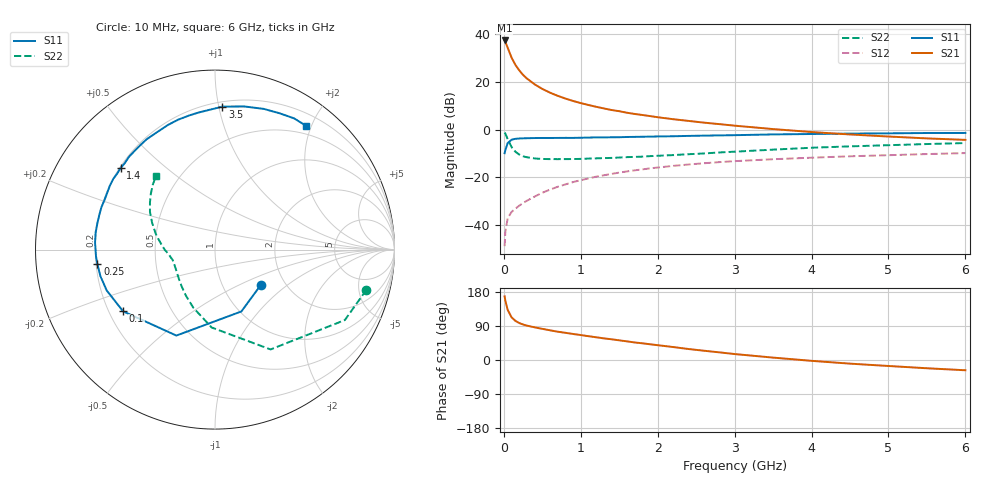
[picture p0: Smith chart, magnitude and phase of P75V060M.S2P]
! SIEMENS Small Signal Semiconductors
! BFP196
! Si NPN RF Bipolar Junction Transistor in SOT143
! VCE = 5 V  IC = 60 mA
! Common Emitter S-Parameters:  May  1996
# GHz  S  MA  R  50
!  f  S11  S21  S12  S22
! GHz  MAG  ANG  MAG  ANG  MAG  ANG  MAG  ANG
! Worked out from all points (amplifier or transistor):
!   36 points, 10 MHz to 6 GHz, reference 50 ohm
!   highest |S21| = 37.5 dB at 10 MHz (marker M1)
!   |S21| within 3 dB of that: start of sweep to 49.2 MHz
!   unconditionally stable (mu >= 1): 442.7 MHz to 4.365 GHz
!   at 250 MHz: K = 0.85, MSG = 26.9 dB, |S12| = -30.8 dB
!   at 1.4 GHz: K = 1.09, MAG = 11.6 dB, |S12| = -18.5 dB
!   at 6 GHz: K = 0.97, MSG = 2.8 dB, |S12| = -9.8 dB
!   S11 on the Smith chart (normalised r, x): 10 MHz: 1.51, -0.67; 100 MHz: 0.26, -0.29; 250 MHz: 0.21, -0.06; 1.4 GHz: 0.20, +0.36; 3.5 GHz: 0.23, +1.03; 6 GHz: 0.37, +1.93
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0.01  0.3225 -37.9  74.82 168.0  0.0036 80.0  0.873 -14.9
0.02  0.3746 -66.9  69.81 156.1  0.0073 70.2  0.823 -28.5
0.05  0.5251 -114.2  52.57 132.3  0.0139 55.4  0.6366 -60.9
0.1  0.6167 -146.1  32.76 112.7  0.0188 48.6  0.4346 -92.4
0.15  0.6449 -159.3  23 103.3  0.022 49.2  0.3454 -110.5
0.2  0.6556 -167.1  17.64 97.6  0.0255 52.9  0.3021 -122.7
0.25  0.6601 -172.9  14.16 93.6  0.0289 55.0  0.2772 -131.9
0.3  0.664 -176.7  11.88 90.7  0.0324 57.7  0.2644 -138.1
0.4  0.6694 176.6  8.989 86.2  0.0395 60.4  0.2497 -147.5
0.5  0.672 171.8  7.197 82.2  0.0476 62.1  0.2436 -153.6
0.6  0.6717 167.3  6 78.4  0.0554 63.2  0.2419 -157.6
0.7  0.673 163.1  5.156 74.7  0.0635 63.0  0.2416 -160.9
0.9  0.6748 155.7  4.016 68.7  0.0797 62.2  0.2426 -165.7
1.1  0.6853 148.8  3.307 62.8  0.0953 60.4  0.248 -168.9
1.4  0.6949 139.0  2.595 54.7  0.1183 56.6  0.2563 -173.0
1.7  0.7084 129.7  2.145 46.3  0.1406 52.5  0.2692 -177.3
2.2  0.7297 116.2  1.665 34.2  0.1743 45.2  0.2936 176.2
2.8  0.761 100.9  1.313 20.2  0.209 36.3  0.3336 166.9
3.5  0.7979 87.0  1.033 6.3  0.2405 26.3  0.3824 156.6
4.5  0.8297 70.9  0.796 -9.6  0.2771 14.4  0.4479 144.0
5.5  0.8538 58.9  0.658 -21.8  0.3087 3.7  0.5011 133.7
6  0.8563 53.5  0.613 -27.1  0.3236 -2.0  0.526 128.7
